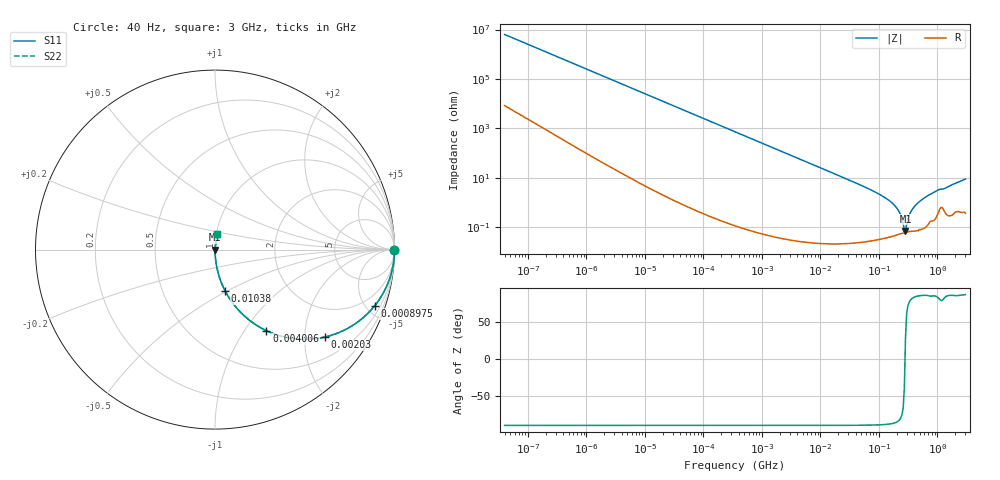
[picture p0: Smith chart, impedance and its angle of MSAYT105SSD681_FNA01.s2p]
! MSAYT105SSD681_FNA01  S-PARAMETER MODEL  ( General Type )
! Model Generated by TAIYO YUDEN Corporation (http://www.ty-top.com)
! Version 2.0
! TAIYO YUDEN Control No. 051115
! Copyright(c) 2005 TAIYO YUDEN CO.,LTD. All Rights Reserved.
! Product Description (link to TY-COMPAS)
! https://ds.yuden.co.jp/TYCOMPAS/or/detail?pn=MSAYT105SSD681KFNA01&u=M
! Products Name : Multilayer Ceramic Capacitors
! Characteristics :
!  Capacitance : 680 pF , Rated Voltage : 25V
!  Case Size : 1.0 x 0.5 / 0.039 x 0.02 [mm/inch] , Thickness : 0.5 / 0.02 [mm/inch]
!  (Conditions: Temperature = 25 degC , DC Bias Current/Voltage = 0A / 0V)
! External Node Assignments :
!  1  o---| |---o  2
! GND o---------o GND
! Frequency Range : 40Hz  -  3GHz  [ 401 STEP ]
# MHz S RI R 50
! Freq[MHz].  S11 Real  S11 Imag  S21 Real  S21 Imag  S12 Real  S12 Imag  S22 Real  S22 Imag
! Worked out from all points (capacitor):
!   401 points, 40 Hz to 3 GHz, reference 50 ohm
!   read as one part in series: C = 627 pF near 44 Hz
!   lowest |Z| = 69.9 mohm at 284 MHz (marker M1)
!   series resonance near 278.9 MHz, so ESL is about 520 pH
!   S11 on the Smith chart (normalised r, x): 40 Hz: open; 897.5 kHz: 1.00, -5.66; 2.03 MHz: 1.00, -2.50; 4.006 MHz: 1.00, -1.27; 10.38 MHz: 1.00, -0.49; 3 GHz: 1.01, +0.18
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4e-05  1 -1.58e-05  2.1e-08 1.58e-05  2.1e-08 1.58e-05  1 -1.58e-05
0.000245  1 -9.65e-05  7.3e-08 9.65e-05  7.3e-08 9.65e-05  1 -9.65e-05
0.000834  1 -0.000328  2.42e-07 0.000328  2.42e-07 0.000328  1 -0.000328
0.017386  1 -0.00685  4.8e-05 0.00685  4.8e-05 0.00685  1 -0.00685
0.362475  0.98 -0.1399  0.02 0.1399  0.02 0.1399  0.98 -0.1399
0.897494  0.8889 -0.3141  0.1111 0.3141  0.1111 0.3141  0.8889 -0.3141
2.029594  0.6102 -0.4876  0.3898 0.4876  0.3898 0.4876  0.6102 -0.4876
4.006119  0.2867 -0.452  0.7133 0.452  0.7133 0.452  0.2867 -0.452
7.222098  0.1101 -0.3127  0.8899 0.3127  0.8899 0.3127  0.1101 -0.3127
10.37922  0.0565 -0.2305  0.9435 0.2305  0.9435 0.2305  0.0565 -0.2305
60.81113  0.00184 -0.0397  0.9982 0.0397  0.9982 0.0397  0.00184 -0.0397
150.5692  0.000536 -0.0119  0.9995 0.0119  0.9995 0.0119  0.000536 -0.0119
206.7996  0.000528 -0.00546  0.9995 0.00546  0.9995 0.00546  0.000528 -0.00546
236.926  0.00056 -0.00294  0.9994 0.00294  0.9994 0.00294  0.00056 -0.00294
259.4108  0.000581 -0.0013  0.9994 0.0013  0.9994 0.0013  0.000581 -0.0013
284.0294  0.000614 0.000334  0.9994 -0.000334  0.9994 -0.000334  0.000614 0.000334
297.2015  0.00062 0.00115  0.9994 -0.00115  0.9994 -0.00115  0.00062 0.00115
340.4975  0.000682 0.00362  0.9993 -0.00362  0.9993 -0.00362  0.000682 0.00362
372.8114  0.000709 0.00536  0.9993 -0.00536  0.9993 -0.00536  0.000709 0.00536
535.7849  0.000997 0.0128  0.999 -0.0128  0.999 -0.0128  0.000997 0.0128
1010.689  0.00436 0.0312  0.9956 -0.0312  0.9956 -0.0312  0.00436 0.0312
3000  0.0114 0.0874  0.9886 -0.0874  0.9886 -0.0874  0.0114 0.0874
